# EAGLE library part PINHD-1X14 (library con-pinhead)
PIN HEADER
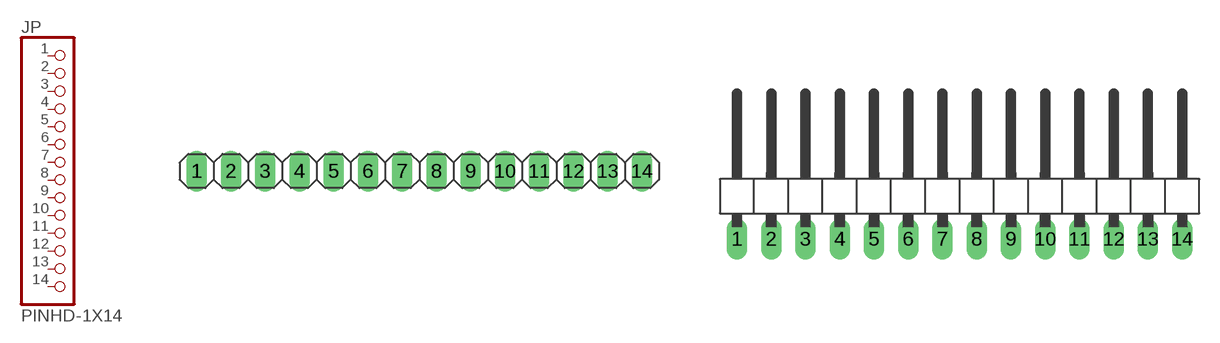
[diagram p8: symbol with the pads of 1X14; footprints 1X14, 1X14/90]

Designator prefix JP

## PINHD-1X14_2.54  [1X14]
1  1  pas
2  2  pas
3  3  pas
4  4  pas
5  5  pas
6  6  pas
7  7  pas
8  8  pas
9  9  pas
10  10  pas
11  11  pas
12  12  pas
13  13  pas
14  14  pas

## PINHD-1X14_2.54-90°  [1X14/90]
Pads as for 1X14

## PINHD-1X14_2.00  [1X14M]
Pads as for 1X14

## PINHD-1X14_2.54-SMD  [1X14SMD]
Pads as for 1X14

## PINHD-1X14_2.54-SMD-90°  [1X14SMD/90]
Pads as for 1X14

## Footprint 1X14 (pad centres in mm)
PIN HEADER - 2.54
drill 1.016 long: 1 -16.51,0; 2 -13.97,0; 3 -11.43,0; 4 -8.89,0; 5 -6.35,0; 6 -3.81,0; 7 -1.27,0; 8 1.27,0; 9 3.81,0; 10 6.35,0; 11 8.89,0; 12 11.43,0; 13 13.97,0; 14 16.51,0

## Footprint 1X14/90 (pad centres in mm)
PIN HEADER - 2.54 90°
drill 1.016 long: 1 -16.51,-3.81; 2 -13.97,-3.81; 3 -11.43,-3.81; 4 -8.89,-3.81; 5 -6.35,-3.81; 6 -3.81,-3.81; 7 -1.27,-3.81; 8 1.27,-3.81; 9 3.81,-3.81; 10 6.35,-3.81; 11 8.89,-3.81; 12 11.43,-3.81; 13 13.97,-3.81; 14 16.51,-3.81

## Footprint 1X14M (pad centres in mm)
PIN HEADER - 2
drill 0.914 square: 1 -13,0
drill 0.914: 2 -11,0; 3 -9,0; 4 -7,0; 5 -5,0; 6 -3,0; 7 -1,0; 8 1,0; 9 3,0; 10 5,0; 11 7,0; 12 9,0; 13 11,0; 14 13,0

## Footprint 1X14SMD (pad centres in mm)
PIN HEADER - 2.54 SMD
smd 1.016 x 3.302: 1 -1.27,1.27; 2 1.27,-1.27; 3 3.81,1.27; 4 6.35,-1.27; 5 8.89,1.27; 6 11.43,-1.27; 7 13.97,1.27; 8 16.51,-1.27; 9 19.05,1.27; 10 21.59,-1.27; 11 24.13,1.27; 12 26.67,-1.27; 13 29.21,1.27; 14 31.75,-1.27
